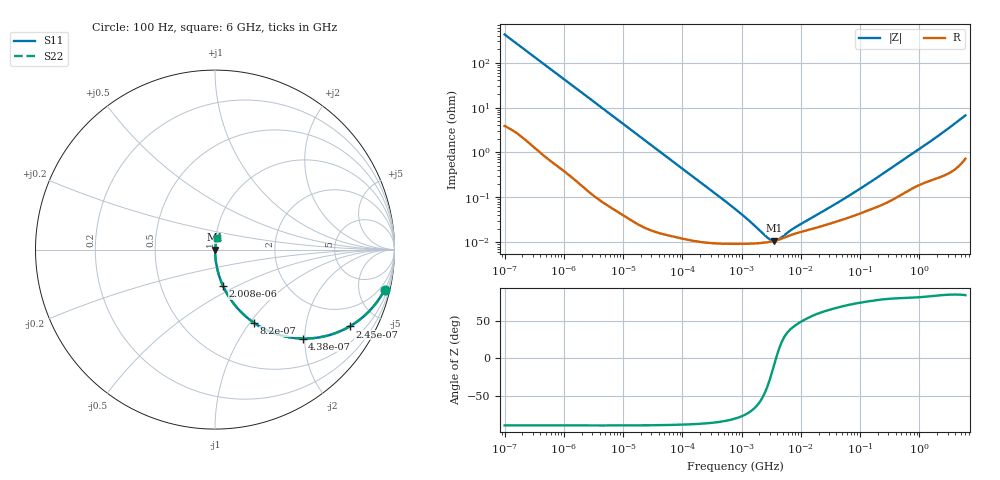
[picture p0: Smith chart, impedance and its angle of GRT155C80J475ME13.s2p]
!Murata Part Number: GRT155C80J475ME13
!These Parameters are Measured in Series Mode Connection
!Data Generated on Jun 19, 2026
!  o--ll--o
!Port1  Port2
!  o------o
!Operation Temp=25[degC], DC Bias Voltage=0[V]
!Freq. Start=100[Hz] Stop=6[GHz] 401[Steps]
# Hz S RI R 50
!Freq.(Hz) S11(Real) S11(Imag) S21(Real) S21(Imag) S12(Real) S12(Imag) S22(Real) S22(Imag)
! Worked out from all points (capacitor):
!   401 points, 100 Hz to 6 GHz, reference 50 ohm
!   read as one part in series: C = 3.75 uF near 109 Hz
!   lowest |Z| = 10.8 mohm at 3.55 MHz (marker M1)
!   series resonance near 3.822 MHz, so ESL is about 460 pH
!   S11 on the Smith chart (normalised r, x): 100 Hz: 1.08, -8.46; 245 Hz: 1.03, -3.48; 438 Hz: 1.02, -1.95; 820 Hz: 1.01, -1.05; 2.008 kHz: 1.00, -0.43; 6 GHz: 1.01, +0.13
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100  0.9453 -0.2229  0.0547 0.2229  0.0547 0.2229  0.9453 -0.2229
164  0.8684 -0.333  0.1316 0.333  0.1316 0.333  0.8684 -0.333
245  0.7499 -0.4281  0.2501 0.4281  0.2501 0.4281  0.7499 -0.4281
335  0.6183 -0.4811  0.3817 0.4811  0.3817 0.4811  0.6183 -0.4811
438  0.4882 -0.4953  0.5118 0.4953  0.5118 0.4953  0.4882 -0.4953
600  0.3396 -0.4691  0.6604 0.4691  0.6604 0.4691  0.3396 -0.4691
820  0.2172 -0.4079  0.7828 0.4079  0.7828 0.4079  0.2172 -0.4079
1227  0.1117 -0.3106  0.8883 0.3106  0.8883 0.3106  0.1117 -0.3106
2008  0.0457 -0.2047  0.9543 0.2047  0.9543 0.2047  0.0457 -0.2047
3437  0.0166 -0.1237  0.9834 0.1237  0.9834 0.1237  0.0166 -0.1237
6433  0.00509 -0.067  0.9949 0.067  0.9949 0.067  0.00509 -0.067
40335  0.000278 -0.0108  0.9997 0.0108  0.9997 0.0108  0.000278 -0.0108
774597  9.2e-05 -0.000546  0.9999 0.000546  0.9999 0.000546  9.2e-05 -0.000546
2713602  9.99e-05 -7.89e-05  0.9999 7.89e-05  0.9999 7.89e-05  9.99e-05 -7.89e-05
3549919  0.000107 -1.63e-05  0.9999 1.63e-05  0.9999 1.63e-05  0.000107 -1.63e-05
4246196  0.000114 2.3e-05  0.9999 -2.3e-05  0.9999 -2.3e-05  0.000114 2.3e-05
7599586  0.000152 0.000137  0.9998 -0.000137  0.9998 -0.000137  0.000152 0.000137
1.555665e7  0.000198 0.000294  0.9998 -0.000294  0.9998 -0.000294  0.000198 0.000294
6.518806e7  0.000356 0.00103  0.9996 -0.00103  0.9996 -0.00103  0.000356 0.00103
3.124326e8  0.000827 0.00414  0.9992 -0.00414  0.9992 -0.00414  0.000827 0.00414
1.637704e9  0.00275 0.0184  0.9972 -0.0184  0.9972 -0.0184  0.00275 0.0184
6e9  0.0115 0.0652  0.9885 -0.0652  0.9885 -0.0652  0.0115 0.0652
